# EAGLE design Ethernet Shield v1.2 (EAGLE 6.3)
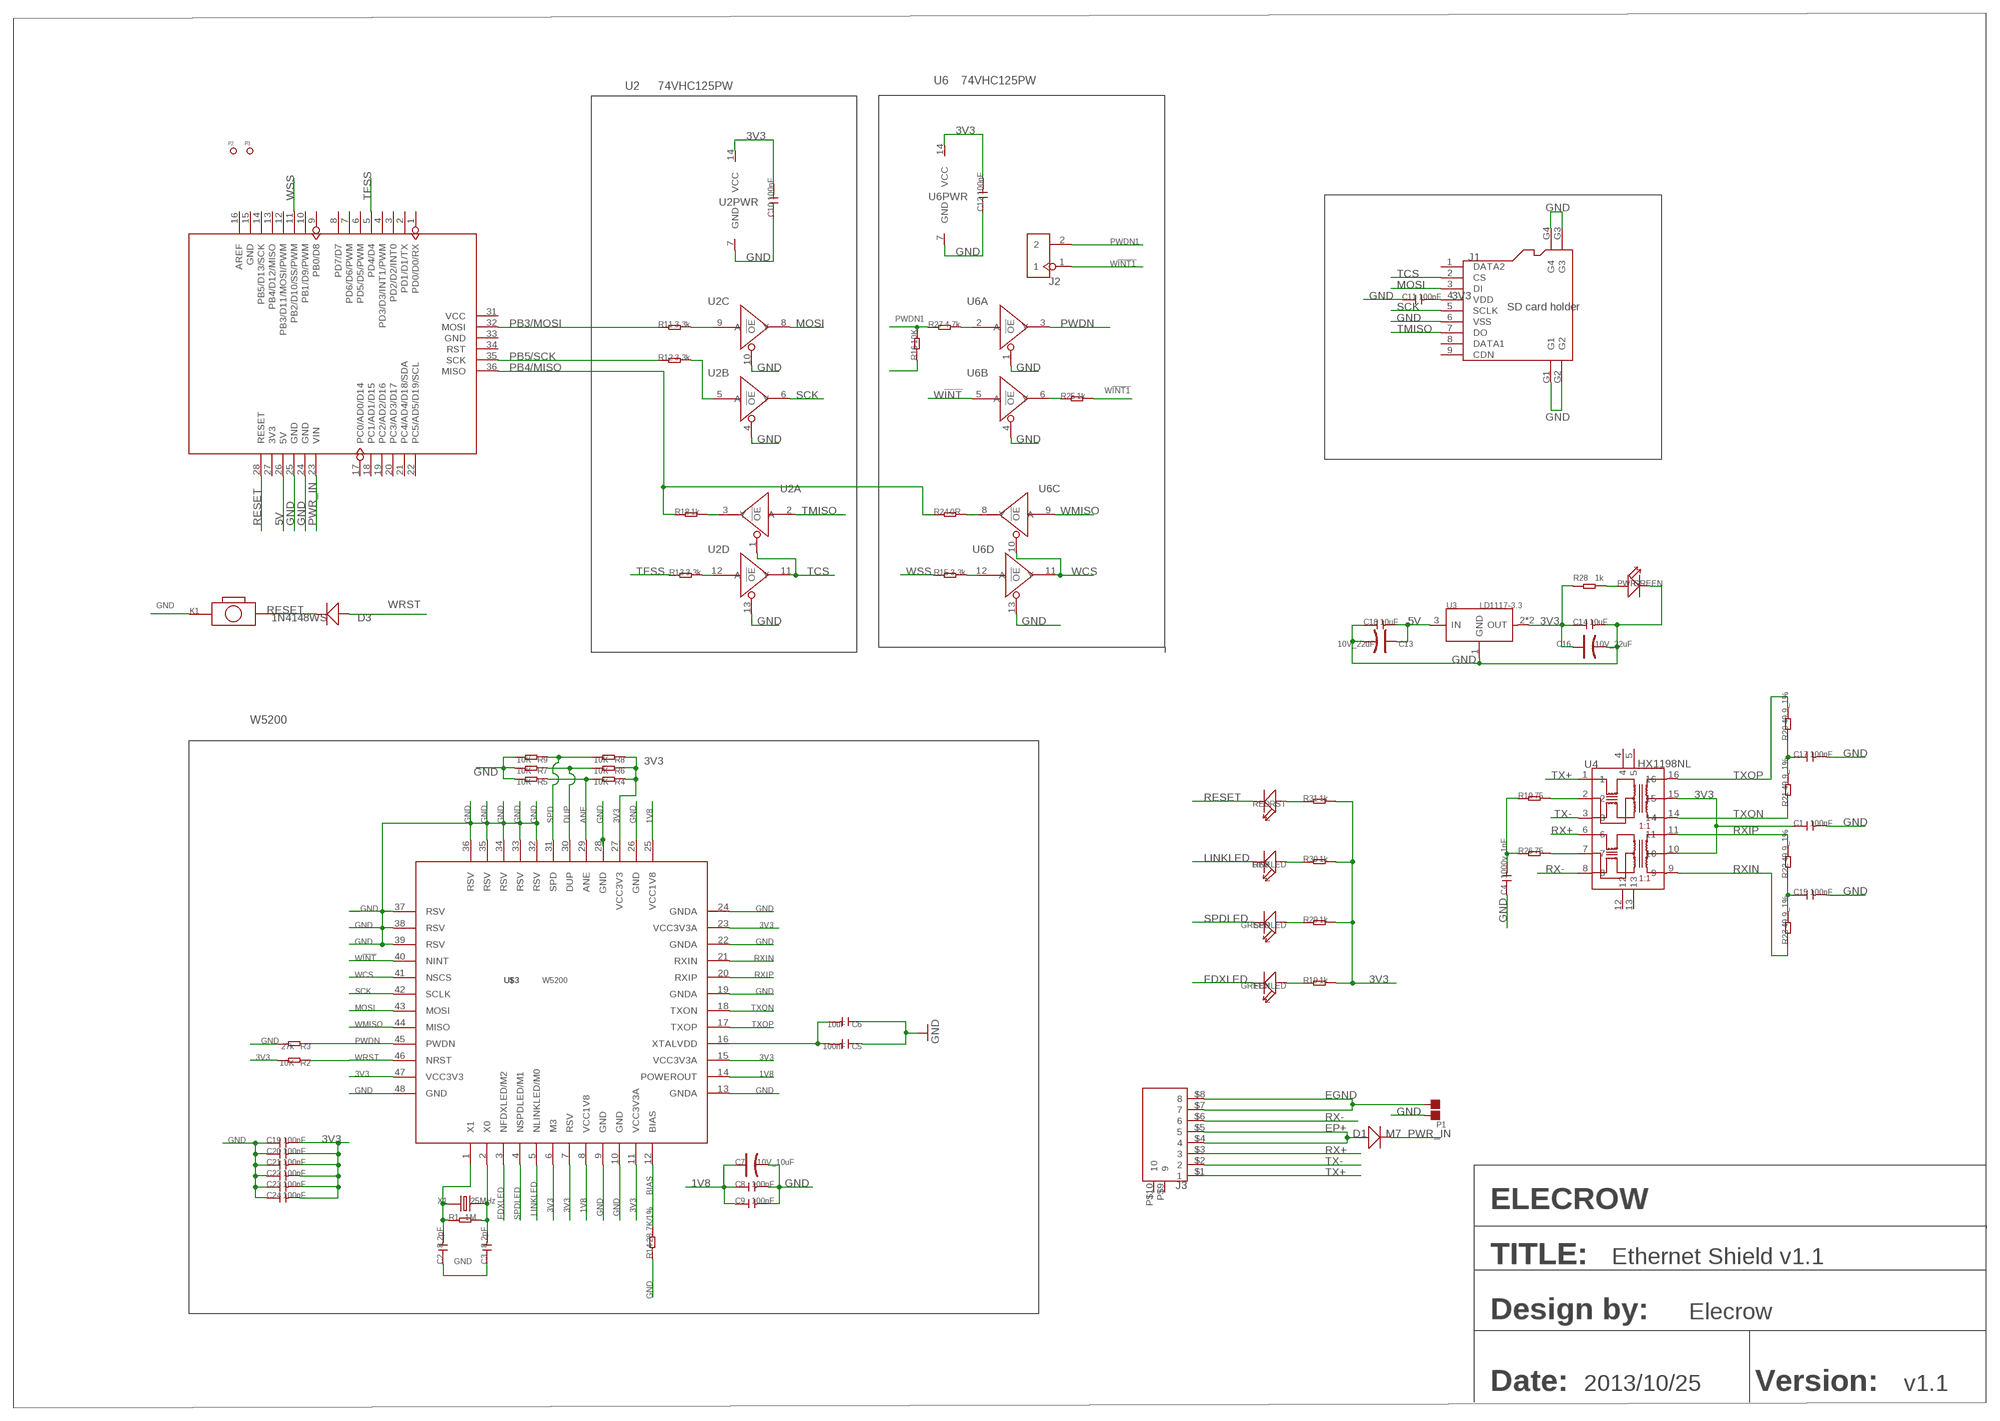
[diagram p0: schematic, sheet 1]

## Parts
C1  100nF  C-0603  [C0603]
C2  8.2pF  C-0603  [C0603]
C3  8.2pF  C-0603  [C0603]
C4  1000v_1nF  C-1206  [C1206]
C5  100nF  C-0603  [C0603]
C6  10uF  C-0805  [C0805]
C7  10V_10uF  CAP-AVX-A  [AVX-A]
C8  100nF  C-0603  [C0603]
C9  100nF  C-0603  [C0603]
C10  100nF  C-0603  [C0603]
C11  100nF  C-0603  [C0603]
C12  100nF  C-0603  [C0603]
C13  10V_22uF  CAP-AVX-B  [AVX-B]
C14  10uF  C-0805  [C0805]
C15  100nF  C-0603  [C0603]
C16  10V_22uF  CAP-AVX-B  [AVX-B]
C17  100nF  C-0603  [C0603]
C18  10uF  C-0805  [C0805]
C19  100nF  C-0805  [C0805]
C20  100nF  C-0805  [C0805]
C21  100nF  C-0805  [C0805]
C22  100nF  C-0805  [C0805]
C23  100nF  C-0805  [C0805]
C24  100nF  C-0805  [C0805]
D1  M7  D'SMA'  [D2010]
D3  1N4148WS  D'0805'  [SOD323]
FDXLED  GREEN  LED'0603'  [LED-0603]
J1  SD card holder  HOLDER-MICROSD-9P  [9P-SMD-W/-RING]
J2  HEADER-2P-65/35MIL  [2P-2.54-65/35MIL]
J3  RJ45-SMD  [RJ45_SMD]
K1  BOTTON-2P-90D  [2P-7.62X3.56-90D]
LINKLED  RED  LED'0603'  [LED-0603]
P1  DNP  PAD-JUMPER-2P  [2P-SMD-1.78X1.27]
P2  PAD-MARK  [ROUND-MARK-1.0]
P3  PAD-MARK  [ROUND-MARK-1.0]
PWR  GREEN  LED'0603'  [LED-0603]
R1  1M  R-0603  [R0603]
R2  10K  R-0603  [R0603]
R3  27k  R-0603  [R0603]
R4  10K  R-0603  [R0603]
R5  10K  R-0603  [R0603]
R6  10K  R-0603  [R0603]
R7  10K  R-0603  [R0603]
R8  10K  R-0603  [R0603]
R9  10K  R-0603  [R0603]
R10  1k  R-0603  [R0603]
R11  3.3k  R-0603  [R0603]
R12  3.3k  R-0603  [R0603]
R13  3.3k  R-0603  [R0603]
R14  28.7K/1%  R-0603  [R0603]
R15  3.3k  R-0603  [R0603]
R16  10K  R-0603  [R0603]
R18  1k  R-0603  [R0603]
R19  75  R-0603  [R0603]
R20  49.9_1%  R-0603  [R0603]
R21  49.9_1%  R-0603  [R0603]
R22  49.9_1%  R-0603  [R0603]
R23  49.9_1%  R-0603  [R0603]
R24  0R  R-0603  [R0603]
R25  1k  R-0603  [R0603]
R26  75  R-0603  [R0603]
R27  4.7k  R-0603  [R0603]
R28  1k  R-0603  [R0603]
R29  1k  R-0603  [R0603]
R30  1k  R-0603  [R0603]
R31  1k  R-0603  [R0603]
RST  RED  LED'0603'  [LED-0603]
SPDLED  GREEN  LED'0603'  [LED-0603]
U1  ARDUINO  [ARDUINO]
U2  74VHC125PW  [TSSOP14]
U3  LD1117-3.3  LD1117S  [SOT-223]
U4  HX1198NL  [SOIC16-9.53]
U6  74VHC125PW  [TSSOP14]
U$3  W5200  [QFN48]
X1  25MHz  CRYSTAL'5032'  [2P-SMD-5X3.2]

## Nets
1V8: C7.+ C8.1 C9.1 U$3.8(VCC1V8) U$3.14(POWEROUT) U$3.25(VCC1V8)
3V3: C1.1 C10.2 C11.2 C12.2 C14.1 C16.+ C19.2 C20.2 C21.2 C22.2 C23.2 C24.2 J1.4(VDD) R2.2 R4.1 R6.1 R8.1 R10.2 R28.1 R29.2 R30.2 R31.2 U2.14(PWR:VCC) U3.2(OUT) U3.TER(OUT) U4.10 U4.15 U6.14(PWR:VCC) U$3.6(M3) U$3.7(RSV) U$3.11(VCC3V3A) U$3.15(VCC3V3A) U$3.23(VCC3V3A) U$3.27(VCC3V3) U$3.47(VCC3V3)
5V [usbvcc]: C13.+ C18.2 U1.26(5V) U3.3(IN)
ANE: R4.2 R5.1 U$3.29(ANE)
BIAS: R14.2 U$3.12(BIAS)
DUP: R6.2 R7.1 U$3.30(DUP)
EGND [power]: J3.$7 J3.$8 P1.1
EP+: D1.+ J3.$4 J3.$5
FDXLED: FDXLED.- U$3.3(NFDXLED/M2)
GND: C1.2 C2.1 C3.1 C4.1 C5.1 C6.1 C7.- C8.2 C9.2 C10.1 C11.1 C12.1 C13.- C14.2 C15.2 C16.- C17.2 C18.1 C19.1 C20.1 C21.1 C22.1 C23.1 C24.1 J1.6(VSS) J1.G1 J1.G2 J1.G3 J1.G4 K1.P$1 P1.2 PWR.- R3.2 R5.2 R7.2 R9.2 R14.1 R16.1 U1.24(GND) U1.25(GND) U2.4(B:!OE) U2.7(PWR:GND) U2.10(C:!OE) U2.13(D:!OE) U3.1(GND) U6.1(A:!OE) U6.4(B:!OE) U6.7(PWR:GND) U6.13(D:!OE) U$3.9(GND) U$3.10(GND) U$3.13(GNDA) U$3.19(GNDA) U$3.22(GNDA) U$3.24(GNDA) U$3.26(GND) U$3.28(GND) U$3.32(RSV) U$3.33(RSV) U$3.34(RSV) U$3.35(RSV) U$3.36(RSV) U$3.37(RSV) U$3.38(RSV) U$3.39(RSV) U$3.48(GND)
LINKLED: LINKLED.- U$3.5(NLINKLED/M0)
MOSI: J1.3(DI) U2.8(C:Y) U$3.43(MOSI)
N$1: R29.1 SPDLED.+
N$2: LINKLED.+ R30.1
N$3: R31.1 RST.+
N$6: FDXLED.+ R10.1
N$7: R12.2 U2.5(B:A)
N$8: R11.2 U2.9(C:A)
N$9: R13.2 U2.12(D:A)
N$10: R15.2 U6.12(D:A)
N$11: R26.2 U4.7
N$12: R19.2 U4.2
N$13: C4.2 R19.1 R26.1
N$14: R18.2 U2.3(A:Y)
N$15: C15.1 R22.1 R23.2
N$16: C17.1 R20.1 R21.2
N$17: R24.2 U6.8(C:Y)
N$20: R25.1 U6.6(B:Y)
N$24: R27.2 U6.2(A:A)
N$26: PWR.+ R28.2
PB3/MOSI: R11.1 U1.32(MOSI)
PB4/MISO: R18.1 R24.1 U1.36(MISO)
PB5/SCK: R12.1 U1.35(SCK)
PWDN: R3.1 U6.3(A:Y) U$3.45(PWDN)
PWDN1: J2.2 R16.2 R27.1
PWR_IN: D1.- U1.23(VIN)
RESET: D3.- K1.P$2 RST.- U1.28(RESET)
RX+: J3.$3 U4.6
RX-: J3.$6 U4.8
RXIN: R23.1 U4.9 U$3.21(RXIN)
RXIP: R22.2 U4.11 U$3.20(RXIP)
SCK: J1.5(SCLK) U2.6(B:Y) U$3.42(SCLK)
SPD: R8.2 R9.1 U$3.31(SPD)
SPDLED: SPDLED.- U$3.4(NSPDLED/M1)
TCS: J1.2(CS) U2.1(A:!OE) U2.11(D:Y)
TFSS: R13.1 U1.5(PD4/D4)
TMISO: J1.7(DO) U2.2(A:A)
TX+: J3.$1 U4.1
TX-: J3.$2 U4.3
TXON: R21.1 U4.14 U$3.18(TXON)
TXOP: R20.2 U4.16 U$3.17(TXOP)
W!INT: U6.5(B:A) U$3.40(NINT)
W!INT1: J2.1 R25.2
WCS: U6.10(C:!OE) U6.11(D:Y) U$3.41(NSCS)
WMISO: U6.9(C:A) U$3.44(MISO)
WRST: D3.+ R2.1 U$3.46(NRST)
WSS: R15.1 U1.11(PB2/D10/SS/PWM)
X0: C3.2 R1.2 U$3.2(X0) X1.2
X1: C2.2 R1.1 U$3.1(X1) X1.1
XTALVDD: C5.2 C6.2 U$3.16(XTALVDD)
Unconnected: J1.1(DATA2) J1.8(DATA1) J1.9(CDN) J3.P$9 J3.P$10 U1.1(PD0/D0/RX) U1.2(PD1/D1/TX) U1.3(PD2/D2/INT0) U1.4(PD3/D3/INT1/PWM) U1.6(PD5/D5/PWM) U1.7(PD6/D6/PWM) U1.8(PD7/D7) U1.9(PB0/D8) U1.10(PB1/D9/PWM) U1.12(PB3/D11/MOSI/PWM) U1.13(PB4/D12/MISO) U1.14(PB5/D13/SCK) U1.15(GND) U1.16(AREF) U1.17(PC0/AD0/D14) U1.18(PC1/AD1/D15) U1.19(PC2/AD2/D16) U1.20(PC3/AD3/D17) U1.21(PC4/AD4/D18/SDA) U1.22(PC5/AD5/D19/SCL) U1.27(3V3) U1.31(VCC) U1.33(GND) U1.34(RST) U4.4 U4.5 U4.12 U4.13

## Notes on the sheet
- U6 | 74VHC125PW
- U2 | 74VHC125PW
- W5200
- ELECROW
- TITLE: | TITLE: | Ethernet Shield v1.1
- Design by: | Elecrow
- Date: | 2013/10/25 | Version: | v1.1

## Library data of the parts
C1-C6 C8-C12 C14 C15 C17-C24 = Discrete:C*: Ceramic Capacitors
C7 C13 C16 = Discrete:CAP*: Electrolytic Capacitors,Tantalum Capacitors and Super Capacitors
D1 D3 = Discrete:D*
FDXLED LINKLED PWR RST SPDLED = Discrete:LED*
J1 = Connector:HOLDER-MICROSD-9P
J2 = Connector:HEADER-2P
J3 = Elecrow_test:RJ45-SMD: Modular Jack 8P8C,R/A,With LED
K1 = Discrete:BOTTON-2P
P1 = Discrete:PAD-JUMPER-2P; PARTNO: DNP
P2 P3 = Discrete:PAD-MARK; PARTNO: DNP
R1-R16 R18-R31 = Discrete:R*
U1 = moudle:ARDUINO
U2 U6 = IC:74V*125: Quad Buffer/Line Driver;3-state
U3 = IC:LD1117: Low Drop Fixed And Adjustable Positive Voltage Regulators http://www.datasheetcatalog.org/datasheet/SGSThomsonMicroelectronics/mXuqtqv.pdf
U4 = IC:HX1198NL: 10/100BASE-T Single Port Surface Mount Magnetics With Various Turns Ratios
U$3 = Elecrow_test:W5200
X1 = Discrete:CRYSTAL*: CRYSTAL

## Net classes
0 default: width 0.203 mm, drill 0.305 mm, clearance 0.152 mm
3 usbvcc: width 0.203 mm, drill 0.305 mm, clearance 0.203 mm

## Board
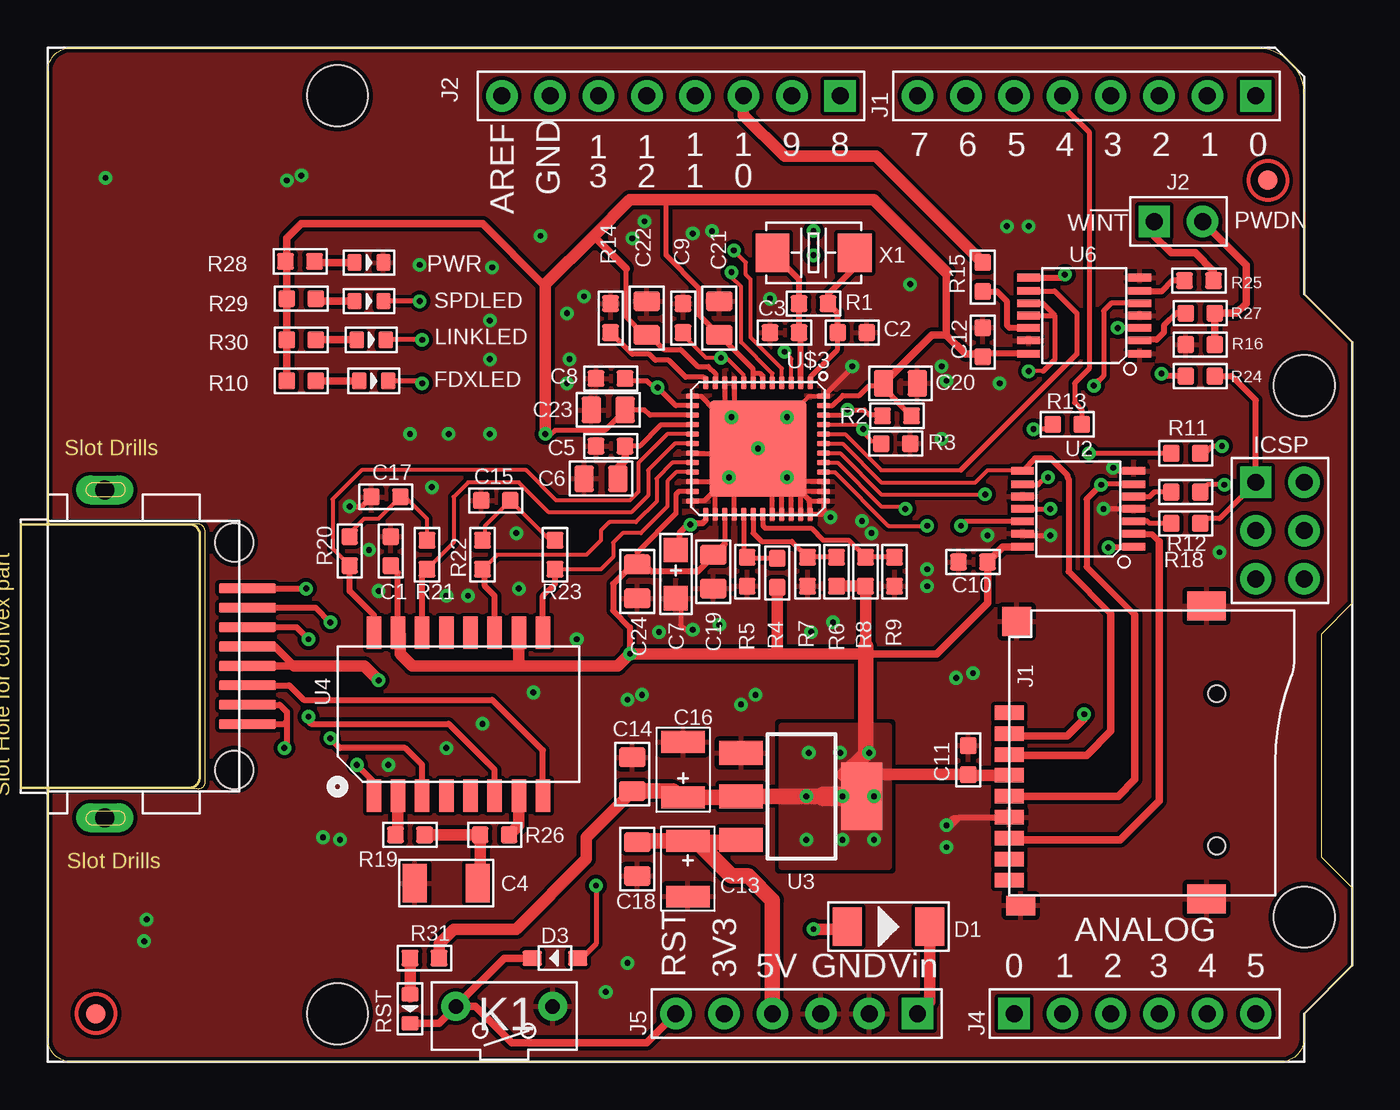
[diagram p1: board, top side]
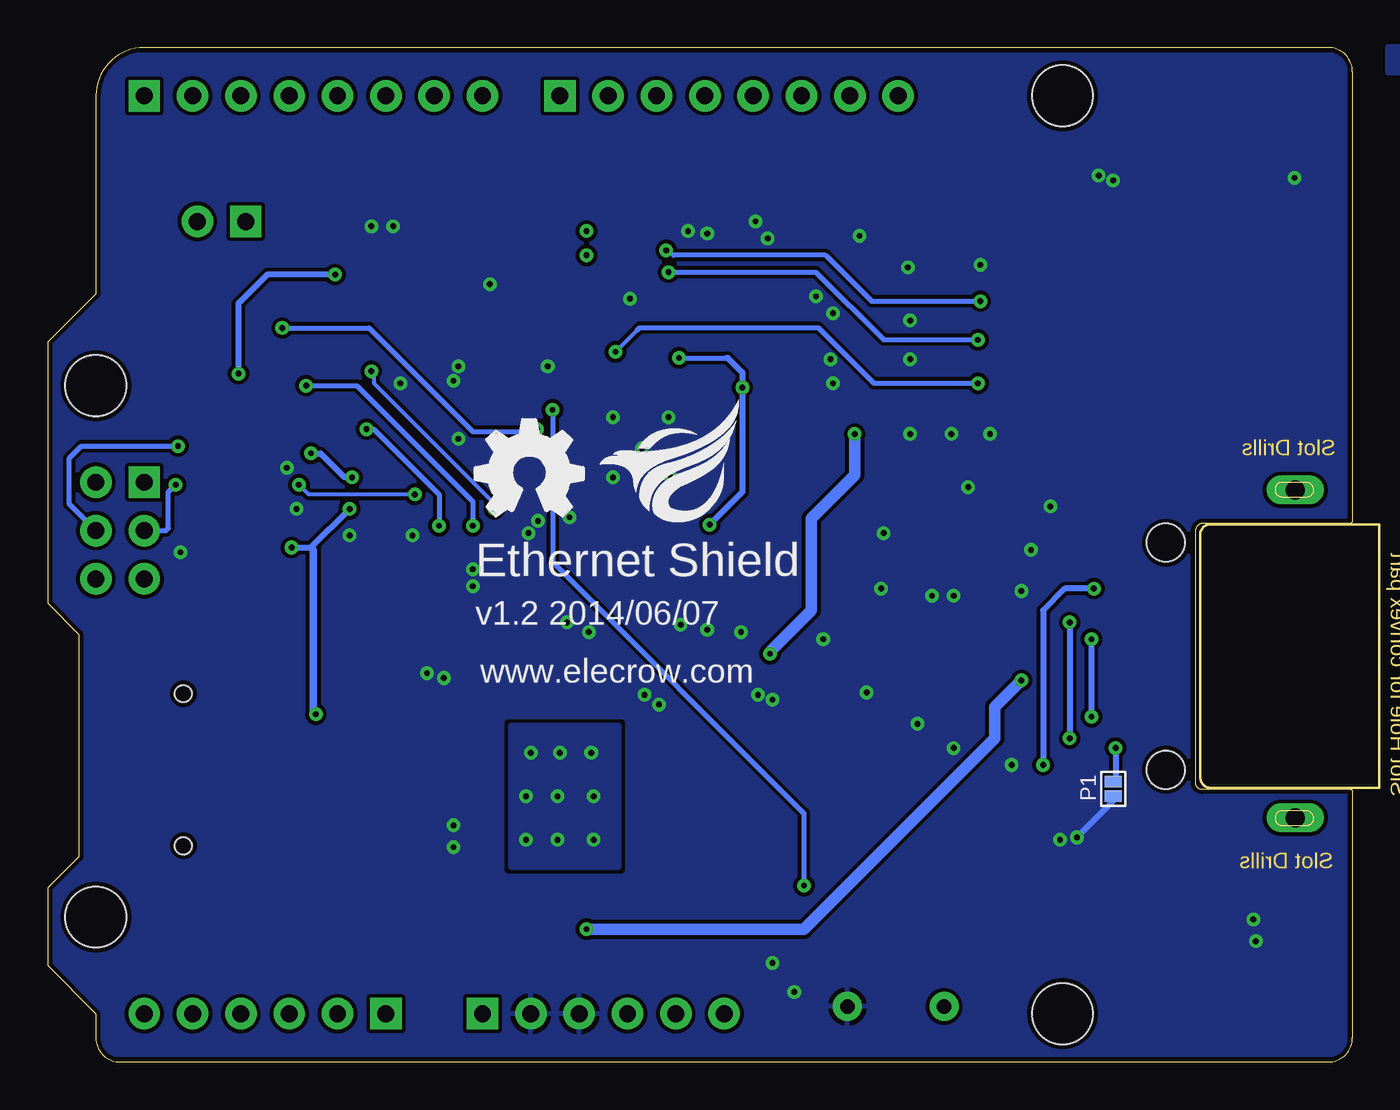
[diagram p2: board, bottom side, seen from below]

Size 68.58 x 53.34 mm. Coordinates in mm from the lower left corner, seen from the top.
Outline: 0,52.07 0,28.45 arc90 0.13,28.32 7.77,28.32 arc-90 8.26,27.96 8.26,14.63 arc-90 7.84,14.35 0.13,14.35 arc90 0,14.22 0,1.27 arc90 1.27,0 64.77,0 arc90 66.04,1.27 66.04,2.54 68.58,5.08 68.58,9.14 66.93,10.79 66.93,22.48 68.58,24.13 68.58,37.85 66.04,40.39 66.04,50.8 arc90 63.5,53.34 1.27,53.34 arc90 0,52.07
Copper layers (1*16): Top 0.035mm / dielectric 1.5mm / Bottom 0.035mm
Design rules "default *": minimum track width 8mil, minimum drill 12mil, track to track 8mil, track to pad 8mil, pad to pad 8mil, via to via 10mil, smd to smd 0mil, copper to edge 10mil, drill to drill 8mil, minimum pad ring 10mil, minimum via ring 8mil, stop-mask expansion 4mil, vias tented up to drill 25mil, thermal gap 10mil
Holes 3.2 mm at 15.24,2.54

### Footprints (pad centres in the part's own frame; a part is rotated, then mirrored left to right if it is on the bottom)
C0603 = smd 0.889 x 0.889: 1 -0.762,0; 2 0.762,0
C1206 = smd 1.27 x 2.032: 1 -1.651,0; 2 1.651,0
C0805 = smd 1.016 x 1.397: 1 -0.889,0; 2 0.889,0
AVX-A = smd 1.27 x 1.27: + -1.27,0; - 1.27,0
AVX-B = smd 1.143 x 2.286: + -1.46,0; - 1.46,0
D2010 = smd 1.524 x 2.032: + -2.159,0; - 2.159,0
SOD323 = smd 1 x 0.8: + -1.2,0; - 1.2,0
LED-0603 = smd 0.762 x 0.889: + -0.762,0; - 0.762,0
9P-SMD-W/-RING = smd 1.524 x 0.762: 1 0,4.4; 2 0,3.3; 3 0,2.2; 4 0,1.1; 5 0,0; 6 0,-1.1; 7 0,-2.2; 8 0,-3.3; 9 0,-4.4 | smd 1.524 x 1.016: G1 0.6,-5.746 | smd 2.032 x 1.524: G2 10.373,-5.4; G3 10.373,10 | smd 1.524 x 1.524: G4 0.392,9.181 | hole 0.889: 10.9,-2.6; 10.9,5.4
2P-2.54-65/35MIL = drill 0.889 pad 1.651 square: 1 0,1.27 | drill 0.889 pad 1.651: 2 0,-1.27
RJ45_SMD = smd 0.5 x 3: $1 -3.57,10.5; $2 -2.55,10.5; $3 -1.53,10.5; $4 -0.51,10.5; $5 0.51,10.5; $6 1.53,10.5; $7 2.55,10.5; $8 3.57,10.5 | drill 1 pad 1.511 long: P$9 8.493,3; P$10 -8.747,3 | hole 2: -5.97,9.8; 5.97,9.8
2P-7.62X3.56-90D = drill 0.762 pad 1.524: P$1 0,2.54; P$2 0,-2.54
2P-SMD-1.78X1.27 = smd 0.889 x 0.61: 1 0,0.381; 2 0,-0.381
ROUND-MARK-1.0 = smd 1.016 x 1.016: P$1 0,0
R0603 = smd 0.889 x 0.889: 1 -0.762,0; 2 0.762,0
ARDUINO = drill 0.889 pad 1.651 square: 1 63.5,50.8; 9 41.656,50.8; 17 50.8,2.54; 23 45.72,2.54; 36 63.5,30.48 | drill 0.889 pad 1.651: 2 60.96,50.8; 3 58.42,50.8; 4 55.88,50.8; 5 53.34,50.8; 6 50.8,50.8; 7 48.26,50.8; 8 45.72,50.8; 10 39.116,50.8; 11 36.576,50.8; 12 34.036,50.8; 13 31.496,50.8; 14 28.956,50.8; 15 26.416,50.8; 16 23.876,50.8; 18 53.34,2.54; 19 55.88,2.54; 20 58.42,2.54; 21 60.96,2.54; 22 63.5,2.54; 24 43.18,2.54; 25 40.64,2.54; 26 38.1,2.54; 27 35.56,2.54; 28 33.02,2.54; 31 66.04,30.48; 32 66.04,27.94; 33 66.04,25.4; 34 63.5,25.4; 35 63.5,27.94 | hole 3.2: 15.24,50.8; 66.04,35.56; 66.04,7.62
TSSOP14 = smd 0.4 x 1.2: 1 -2,-2.925; 2 -1.3,-2.925; 3 -0.65,-2.925; 4 0,-2.925; 5 0.65,-2.925; 6 1.3,-2.925; 7 2,-2.925; 8 2,2.925; 9 1.3,2.925; 10 0.65,2.925; 11 0,2.925; 12 -0.65,2.925; 13 -1.3,2.925; 14 -2,2.925
SOT-223 = smd 1.27 x 2.286: 1 -2.286,-3.175; 2 0,-3.175; 3 2.286,-3.175 | smd 3.556 x 2.159: TER 0,3.175
SOIC16-9.53 = smd 0.762 x 1.714: 1 -4.445,-4.286; 2 -3.175,-4.286; 3 -1.905,-4.286; 4 -0.635,-4.286; 5 0.635,-4.286; 6 1.905,-4.286; 7 3.175,-4.286; 8 4.445,-4.286; 9 4.445,4.286; 10 3.175,4.286; 11 1.905,4.286; 12 0.635,4.286; 13 -0.635,4.286; 14 -1.905,4.286; 15 -3.175,4.286; 16 -4.445,4.286
QFN48 = smd 0.3 x 0.7: 1 -2.369,-2.815; 2 -1.869,-2.815; 3 -1.369,-2.815; 4 -0.869,-2.815; 5 -0.369,-2.815; 6 0.131,-2.815; 7 0.631,-2.815; 8 1.131,-2.815; 9 1.631,-2.815; 10 2.131,-2.815; 11 2.631,-2.815; 12 3.131,-2.815; 25 3.131,4.085; 26 2.631,4.085; 27 2.131,4.085; 28 1.631,4.085; 29 1.131,4.085; 30 0.631,4.085; 31 0.131,4.085; 32 -0.369,4.085; 33 -0.869,4.085; 34 -1.369,4.085; 35 -1.869,4.085; 36 -2.369,4.085 | smd 0.7 x 0.3: 13 3.831,-2.115; 14 3.831,-1.615; 15 3.831,-1.115; 16 3.831,-0.615; 17 3.831,-0.115; 18 3.831,0.385; 19 3.831,0.885; 20 3.831,1.385; 21 3.831,1.885; 22 3.831,2.385; 23 3.831,2.885; 24 3.831,3.385; 37 -3.069,3.385; 38 -3.069,2.885; 39 -3.069,2.385; 40 -3.069,1.885; 41 -3.069,1.385; 42 -3.069,0.885; 43 -3.069,0.385; 44 -3.069,-0.115; 45 -3.069,-0.615; 46 -3.069,-1.115; 47 -3.069,-1.615; 48 -3.069,-2.115 | smd 5.1 x 5.1: PAD 0.381,0.635
2P-SMD-5X3.2 = smd 1.778 x 2.032: 1 -2.159,0; 2 2.159,0

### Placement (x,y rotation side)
C1  18.03,26.86 90 top
C2  42.29,38.35 180 top
C3  38.73,38.35 0 top
C4  20.95,9.4 0 top
C5  29.59,32.38 0 top
C6  29.08,30.67 0 top
C7  33.02,25.65 270 top
C8  29.59,35.94 180 top
C9  33.4,39.12 90 top
C10  48.64,26.29 0 top
C11  48.39,15.88 270 top
C12  49.15,37.85 270 top
C13  33.66,10.16 270 top
C14  30.73,15.14 90 top
C15  23.56,29.53 180 top
C16  33.4,15.37 90 top
C17  17.78,29.72 180 top
C18  30.99,10.67 90 top
C19  34.99,25.78 90 top
C20  44.83,35.69 180 top
C21  35.31,39.12 270 top
C22  31.5,39.12 270 top
C23  29.46,34.29 0 top
C24  30.99,25.27 90 top
D1  44.2,7.11 0 top
D3  26.67,5.46 180 top
FDXLED  17.14,35.81 0 top
J1  50.55,13.97 0 top
J2  59.44,44.2 90 top
J3  0,21.34 270 top
K1  24,2.92 270 top
LINKLED  17.02,37.97 0 top
P1  12.57,14.35 0 bottom
P2  2.54,2.54 0 top
P3  64.14,46.35 0 top
PWR  16.89,42.04 0 top
R1  40.26,39.88 180 top
R2  44.64,33.97 0 top
R3  44.58,32.51 0 top
R4  38.35,25.72 90 top
R5  36.77,25.78 270 top
R6  41.47,25.78 90 top
R7  39.94,25.78 270 top
R8  42.99,25.78 90 top
R9  44.51,25.78 270 top
R10  13.34,35.81 180 top
R11  59.82,32 180 top
R12  59.82,29.97 180 top
R13  53.59,33.53 180 top
R14  29.59,39.12 270 top
R15  49.15,41.27 270 top
R16  60.58,37.72 0 top
R18  59.82,28.32 180 top
R19  19.05,11.94 180 top
R20  15.88,26.86 270 top
R21  19.94,26.67 90 top
R22  22.86,26.67 270 top
R23  26.67,26.67 90 top
R24  60.58,36.07 180 top
R25  60.52,41.08 0 top
R26  23.5,11.94 0 top
R27  60.58,39.37 180 top
R28  13.27,42.1 0 top
R29  13.34,40.13 180 top
R30  13.34,37.97 180 top
R31  19.81,5.46 0 top
RST  19.05,2.79 270 top
SPDLED  16.89,40.01 0 top
U1  0,0 0 top
U2  54.17,29.08 90 top
U3  39.62,13.97 270 top
U4  21.59,18.29 0 top
U6  54.48,39.24 90 top
U$1  [ELECROW_NRW_6]  39.56,28.38 0 bottom
U$2  [OSHW_FILLX200_NOTEXT]  46.1,28.7 0 bottom
U$3  37.72,32.89 180 top
X1  40.26,42.55 180 top

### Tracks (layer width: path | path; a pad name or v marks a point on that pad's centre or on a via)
1V8  (via drill 0.3)
  Top 0.203: U$3.8 36.59,36.12 35.69,37.02 v35.4,37.02 34.61,37.02 33.4,38.23 C9.1
  Top 0.254: C8.1 30.48,35.81 31.5,35.81 31.85,35.46 v32.07,35.46 33.02,34.51 U$3.14 | U$3.25 34.59,28.49
  Top 0.305: 34.59,28.49 34.42,28.32 33.85,28.32 v33.78,28.26 33.66,28.26 33.21,27.81 33.21,27.11 C7.+
  Bottom 0.254: v35.4,37.02 32.89,37.02
  Bottom 0.305: 32.89,37.02 32.83,37.02 32.07,36.26 v32.07,35.46 32.07,29.97 v33.78,28.26
3V3  (via drill 0.3)
  Top 0.254: U$3.6 37.59,36.07 37.47,36.2 37.09,36.2 | U$3.7 37.09,36.2 | 37.09,36.2 37.09,36.45 C21.2 34.23,39.31 34.23,40.7 32.51,42.42 32.51,45.34 | U$3.23 33.18,30.01 33.02,29.84 33.02,28.83 30.99,26.8 C24.2 30.99,26.42 31.11,26.54 | 30.67,33.97 30.61,34.04 | 30.61,34.04 C23.2 | U$3.27 35.59,27.27 C19.2 | R2.2 43.94,35.43 C20.2 43.81,35.56 43.18,35.56 42.67,35.05 41.78,35.05 41.24,34.51 U$3.47 | 30.61,34.04 30.61,33.78 | 26.29,33.15 v26.16,33.02 26.48,33.02 26.67,33.21 29.27,33.21 C23.2 | C23.2 31.37,34.29 31.65,34.01 U$3.15 | 31.75,25.78 31.37,26.16 | 26.29,39.12 26.16,39.24 | 30.42,41.72 30.42,39.18 31.37,38.23 C22.2 31.62,38.23 32.38,37.47 33.27,37.47 34.16,36.58 34.73,36.58 35.12,36.2 35.12,35.74 U$3.11 35.05,35.74
  Top 0.305: U6.14 49.31,37.24 C12.2 49.02,36.96 | 35.59,27.27 35.59,27.21 34.16,25.78 31.75,25.78 | 31.37,26.54 31.11,26.54 29.72,25.15 29.72,23.75 30.61,22.86 v30.61,21.46 | U4.15 18.41,25.72 C1.1 | 31.37,26.16 C24.2
  Top 0.406: 30.42,41.72 28.7,43.43 | 47.24,41.53 47.24,38.23 | 47.24,38.23 48.26,37.21 49.02,37.21 C12.2 | 47.24,38.23 46.48,38.23 C20.2 | 26.16,40.89 26.04,40.89 22.86,44.07 13.34,44.07 12.57,43.31 12.57,42.16 R28.1 12.57,42.04 R29.2 R30.2 R10.2 | U2.14 50.2,27.08 C10.2 49.4,24.13 46.74,21.46 43.18,21.46
  Top 0.61: 38.35,21.46 43.18,21.46 42.99,21.65 42.99,21.84 R8.1 R6.1 | 38.35,21.46 v30.61,21.46 29.97,20.83 24.77,20.83 | R4.1 38.35,21.46 | U4.15 18.54,22.45 18.54,21.46 19.18,20.83 24.77,20.83 | U4.10 24.77,20.83 | J1.4 48.43,15.07 C11.2 41.91,15.11 | v26.16,33.02 26.16,39.24 26.16,40.89 28.7,43.43 30.61,45.34 32.51,45.34 43.43,45.34 47.24,41.53 | C14.1 30.73,14.22 28.32,11.81 28.32,10.67 24.64,6.99 21.34,6.99 20.57,6.22 R31.2
  Top 0.813: 41.91,15.11 42.99,16.19 42.99,21.84 | 40.77,13.97 v39.88,13.97 U3.2 36.39,13.91 C16.+ 33.34,13.97 32.77,13.97 32.89,13.84 33.27,13.84 32.87,14.25 C14.1
  Top 1.016: 40.77,13.97 U3.TER
  Bottom 0.61: v30.61,21.46 30.61,21.59 28.45,23.75 28.45,28.57 26.16,30.86 v26.16,33.02
  other vias: 40.01,16.26 39.88,11.68 41.78,11.68 43.43,11.68 41.78,13.97 43.43,13.97 41.66,16.26 43.18,16.26
  pour Top (isolate 0.406, no thermals): 38.61,10.29 44.2,10.29 44.2,17.65 38.61,17.65
  pour Bottom (isolate 0.406, no thermals): 38.61,10.29 44.2,10.29 44.2,17.65 38.61,17.65
5V
  Top 0.813: U1.26 38.1,8.51 36.83,9.78 35.94,9.78 34.16,11.56 33.72,11.56 C13.+ | C13.+ 34.35,11.62 34.42,11.56 36.32,11.56 U3.3 | C13.+ 31.05,11.62 C18.2
ANE
  Top 0.254: 36.52,26.79 R5.1 | U$3.29 36.59,26.72 R5.1 | R4.2 36.83,26.48 R5.1
BIAS
  Top 0.254: U$3.12 34.59,35.9 34.48,36.01 33.53,36.01 32.64,36.89 31.94,36.89 31.62,37.21 30.73,37.21 R14.2
DUP
  Top 0.254: U$3.30 37.09,27.81 37.53,27.37 39.12,27.37 R7.1 R6.2
EGND  (via drill 0.3)
  Top 0.305: J3.$8 12.43,17.77 12.57,17.91 | J3.$7 12.2,18.79 12.57,18.41 12.57,17.91 | 12.57,17.91 12.57,16.64 v12.45,16.51
  Bottom 0.305: v12.45,16.51 12.45,14.86 P1.1
EP+  (via drill 0.3)
  Top 0: v17.4,20.07 v17.39,20.07
  Top 0.406: J3.$5 12.95,20.83 11.93,21.85 J3.$4 | 16.64,20.83
  Top 0.61: D1.+ 41.91,6.99 v40.26,6.99 | 12.95,20.83 16.64,20.83 v17.4,20.07
  Bottom 0.61: v40.26,6.99 28.83,6.99 18.8,17.02 18.8,18.67 v17.4,20.07
FDXLED  (via drill 0.3)
  Top 0.203: U$3.3 39.09,36.98 v38.73,37.34
  Top 0.254: v19.68,35.69 19.56,35.81 FDXLED.-
  Bottom 0.203: v38.73,37.34 37.59,38.48
  Bottom 0.254: 37.59,38.48 37.47,38.61 28.07,38.61 25.15,35.69 v19.68,35.69
GND  (via drill 0.3)
  Top 0.203: U$3.48 40.77,34.99 40.01,34.99 38.92,33.91 v38.86,33.91
  Top 0.254: v38.86,33.91 38.99,33.91 | U$3.48 42.29,36.51 v42.29,36.58 | v15.88,29.21 16.51,29.21 C17.2 | U$3.9 36.09,33.91 v35.94,33.91 35.59,34.26 | U$3.10 35.59,34.26 | U$3.13 34.33,35.01 35.05,34.29 35.56,34.29 35.59,34.26 | U$3.22 35.59,30.51 v35.81,30.73 | U$3.26 35.09,30.01 | 35.09,30.01 v35.81,30.73 | U$3.28 36.09,30.73 v35.81,30.73 | U$3.32 38.09,29.96 v38.86,30.73 | U$3.33 38.59,30.46 v38.86,30.73 | U$3.34 39.09,30.51 | U$3.35 39.59,30.01 | 39.59,30.01 v38.86,30.73 | U$3.38 39.59,30.01 | U$3.39 39.09,30.51 | 39.09,30.51 v38.86,30.73 | v38.86,30.73 40.07,29.53 | 40.07,29.53 40.09,29.51 U$3.37 40.79,29 v41.15,28.64 40.98,28.81 U$3.36 40.07,28.83 40.07,29.53 | 35.09,30.01 34.96,30.01 34.96,29.95 34.54,29.53 33.91,29.53 U$3.24 | U2.4 v55.5,29.08 | U2.13 51.34,27.69 v52.7,27.69 | C7.- 33.27,24.13 33.27,22.99 33.53,22.73 v33.91,22.73 | U$3.19 36.2,32 36.45,32.26 v37.34,32.26 | U2.7 56.17,31.08 v56.01,31.24
  Top 0.305: J1.6 50.5,12.83 47.88,12.83 | 47.88,12.83 47.5,12.45 v47.24,12.45 47.62,12.83 47.88,12.83
  Bottom 0.305: P1.2 12.57,13.72 v14.48,11.81
  other vias: 46.99,36.58 47.24,35.81 42.8,28.45 43.31,27.81 46.23,25.91 46.23,25.02 41.27,23.11 40.13,22.61 35.31,22.99 15.37,11.68 23.24,36.96 19.05,33.02 21.08,33.02 31.37,44.2 30.73,43.31 28.19,40.26 27.3,39.37 27.43,36.96 27.3,35.69 20.95,24.51 22.1,24.51 20.19,30.23 17.4,24.77 17.91,15.62 29.34,3.68 30.48,5.21 16.89,26.92 23.24,33.02 30.48,19.05 31.24,19.3 20.95,16.51 22.86,17.78 25.53,19.43 47.24,11.3 47.75,20.19 48.64,20.45 46.99,32.77 50.04,35.69 33.91,43.56 34.92,43.69 45.34,40.89 37.97,40.13 32.13,22.61 23.24,38.99 23.37,41.78 19.56,41.91 5.21,7.49 3.05,46.48 37.21,19.3 5.08,6.35 13.34,46.61 36.45,18.8 61.59,26.8 50.42,43.94 51.56,43.94 25.91,43.43 12.57,46.35 49.4,27.69 24.77,24.89 24.64,27.81 27.81,22.23
  pour Bottom: -3.17,53.34 -1.91,53.34 -1.91,52.07 -3.17,52.07
  pour Top (rank 6): 0,53.34 68.96,53.34 68.96,0 68.96,-0.13 0,-0.13
  pour Bottom (isolate 0.152, rank 6): 0,53.34 68.83,53.34 68.83,-0.13 0,-0.13
LINKLED  (via drill 0.3)
  Top 0.203: U$3.5 38.09,36.21 36.45,37.85 36.45,40.77 35.94,41.27 v35.94,41.53
  Top 0.254: v19.68,37.97 LINKLED.-
  Bottom 0.254: v19.68,37.97 24.64,37.97 28.19,41.53 v35.94,41.53
MOSI
  Top 0.203: U$3.43 41.79,32.51 43.81,30.48 48.77,30.48 49.4,31.11 50.16,31.11 50.67,31.11 51.21,31.11 U2.8
  Top 0.305: U2.8 51.91,31.75 52.7,31.75 53.59,30.86 53.59,30.73 53.66,30.67 53.66,25.78 55.88,23.56
  Top 0.406: J1.3 50.59,16.13 54.61,16.13 55.88,17.4 55.88,23.56
N$1
  Top 0.406: R29.1 14.22,40.01 SPDLED.+
N$2
  Top 0.406: R30.1 LINKLED.+
N$3
  Top 0.61: R31.1 RST.+ 19.05,3.43
N$6
  Top 0.406: R10.1 FDXLED.+
N$7
  Top 0.254: R12.2 58.17,29.97 57.91,29.72 57.1,29.72 U2.5
N$8  (via drill 0.3)
  Top 0.254: R11.2 v54.74,32 | U2.9 51.27,30.35 52.07,30.35 52.45,30.73 v52.58,30.73
  Bottom 0.305: v54.74,32 54.23,32 52.96,30.73 v52.58,30.73
N$9  (via drill 0.3)
  Top 0.254: 51.23,28.45 U2.12 48.24,28.43 v48.01,28.19 | R13.2 52.58,33.27 v51.82,33.27
  Bottom 0.254: v51.82,33.27 51.44,33.27 48.01,29.84 v48.01,28.19
N$10
  Top 0.305: R15.2 49.91,40.51 50.42,40.01 50.42,38.73 50.55,38.61 51.54,38.61 U6.12
N$11
  Top 0.61: U4.7 24.77,12.45 R26.2
N$12
  Top 0.61: U4.2 18.41,12.06 R19.2
N$13
  Top 0.61: R19.1 R26.1 22.73,9.53 C4.2
N$14
  Top 0.254: R18.2 57.91,28.32 57.78,28.45 57.1,28.45 U2.3
N$15
  Top 0.203: R23.2 26.42,27.43 C15.1 22.99,28.19 22.99,27.56 R22.1
N$16
  Top 0.203: R20.1 15.88,27.81 16.64,28.57 17.4,28.57 C17.1 18.8,29.72 19.94,28.57 R21.2
N$17  (via drill 0.3)
  Top 0.305: U6.8 53.31,41.24 v53.47,41.4 | R24.2 58.67,36.07 v58.55,36.2
  Bottom 0.305: v53.47,41.4 57.02,41.4 58.55,39.88 v58.55,36.2
N$20
  Top 0.305: R25.1 59.12,41.08 58.55,40.51 57.44,40.51 U6.6
N$21  (via drill 0.3)
  other vias: 40.26,43.69
N$22  (via drill 0.3)
  other vias: 40.26,42.42
N$24
  Top 0.305: R27.2 59.31,39.37 58.67,38.73 58.67,38.35 58.29,37.97 57.44,37.97 U6.2
N$26
  Top 0.406: R28.2 14.1,42.04 PWR.+
PB3/MOSI  (via drill 0.3)
  Top 0.254: 61.34,32.38 v61.72,32.38 61.21,32.38 60.83,32 R11.1
  Bottom 0.254: U1.32 67.44,29.34 67.44,31.75 66.8,32.38 v61.72,32.38
PB4/MISO
  Top 0.254: U1.36 61.59,28.57 60.83,28.57 R18.1
  Top 0.305: U1.36 63.5,34.8 62.23,36.07 R24.1
PB5/SCK  (via drill 0.3)
  Top 0.254: v61.85,30.35 60.96,30.35 R12.1
  Bottom 0.254: U1.35 62.36,27.94 62.23,28.07 62.23,29.97 v61.85,30.35
PWDN  (via drill 0.3)
  Top 0.203: U$3.45 42.63,33.51 v42.86,33.27 42.86,33.08 43.31,32.64 43.69,32.64
  Top 0.254: R3.1 43.69,32.64
  Top 0.305: U6.3 v56.25,38.59
  Bottom 0.203: 42.99,33.15 v42.86,33.27
  Bottom 0.254: v56.25,38.59 51.67,38.59 46.23,33.15 42.99,33.15
PWDN1
  Top 0.406: J2.2 62.99,41.91 62.99,39.88 62.48,39.37 R27.1 R16.2
PWR_IN
  Top 0.61: U1.23 46.35,3.17 D1.-
RESET
  Top 0.406: 20.95,2.41 K1.P$2 | K1.P$2 22.48,2.92 24.38,1.02 31.5,1.02 U1.28 32.89,2.67 | D3.- 24,5.46 K1.P$2 | RST.- 20.57,2.03 K1.P$2
RX+  (via drill 0.3)
  Top 0.305: U4.6 23.5,15.37 21.08,17.78 13.84,17.78 13.72,17.91 v13.72,18.16 | J3.$3 13.07,22.87 v13.72,22.23
  Bottom 0.305: v13.72,22.23 v13.72,18.16
RX-
  Top 0.305: U4.8 26.04,16.38 23.37,19.05 13.46,19.05 12.7,19.81 12.69,19.81 J3.$6
RXIN
  Top 0.203: U$3.21 33.04,31.01 32.58,30.54 32.58,29.21 31.18,27.81 30.23,27.81 29.72,27.3 29.72,26.54 29.08,25.91 R23.1
  Top 0.305: U4.9 26.04,24.51 26.67,25.15 R23.1
RXIP
  Top 0.203: U$3.20 32.84,31.51 32,30.67 32,29.46 30.92,28.38 29.53,28.38 29.08,27.94 29.08,27.43 28.32,26.67 23.62,26.67 R22.2
  Top 0.305: U4.11 23.5,24.51 22.99,25.02 22.99,25.78 R22.2
SCK  (via drill 0.3)
  Top 0.203: U$3.42 41.65,32.01 43.81,29.84 v49.28,29.84
  Top 0.254: U2.6 55.4,30.38 v55.37,30.35
  Top 0.305: 57.15,23.5 54.61,26.04 54.61,29.59 v55.37,30.35
  Top 0.406: J1.5 56.26,13.97 57.15,14.86 57.15,23.5
  Bottom 0.203: v49.28,29.84 54.86,29.84 v55.37,30.35
SPD
  Top 0.254: U$3.31 37.59,28.2 37.72,28.07 40.13,28.07 40.77,27.43 42.1,27.43 R8.2 R9.1
SPDLED  (via drill 0.3)
  Top 0.203: U$3.4 38.59,36.47 36.96,38.1 36.96,41.15 36.7,41.4 36.7,42.04 v36.07,42.67
  Top 0.254: v19.56,40.01 SPDLED.-
  Bottom 0.203: 35.69,42.42 35.94,42.67 v36.07,42.67
  Bottom 0.254: v19.56,40.01 25.27,40.01 27.69,42.42 35.69,42.42
TCS  (via drill 0.3)
  Top 0.254: U2.11 v52.7,29.08
  Top 0.305: U2.1 56.04,27.08 56.01,27.05 v55.75,27.05
  Top 0.406: J1.2 50.67,17.14 53.59,17.14 54.48,18.03 v54.48,18.29
  Bottom 0.305: v52.7,29.08 54.74,27.05 | v55.75,27.05 54.74,27.05 | 54.74,27.05 54.61,26.92
  Bottom 0.406: v54.48,18.29 54.61,18.41 54.61,26.92
TFSS
  Top 0.254: U1.5 53.34,50.29 54.74,48.9 54.74,36.45 53.98,35.69 53.98,34.67 54.36,34.29 R13.1
TMISO
  Top 0.305: U2.2 57.12,27.75 58.04,27.75 58.42,27.37
  Top 0.406: J1.7 50.63,11.68 56.39,11.68 58.42,13.72 58.42,27.37
TX+  (via drill 0.3)
  Top 0.254: 17.14,13.72 17.4,13.46 17.4,13.75 U4.1
  Top 0.305: 10.51,24.89 J3.$1 13.57,24.91 v13.59,24.89 | v16.26,15.62 17.14,14.73 U4.1
  Bottom 0.305: v13.59,24.89 15.11,24.89 16.26,23.75 v16.26,15.62
TX-  (via drill 0.3)
  Top 0.305: U4.3 19.68,15.62 18.8,16.51 15.37,16.51 v14.86,17.02 | J3.$2 14.09,23.89 v14.86,23.11
  Bottom 0.305: v14.86,23.11 v14.86,17.02
TXON
  Top 0.203: U$3.18 32.95,32.51 31.56,31.11 31.56,29.78 30.67,28.89 26.35,28.89 24.77,30.48 22.1,30.48 21.34,29.72 21.34,27.3 R21.1
  Top 0.305: U4.14 19.68,25.65 R21.1
TXOP
  Top 0.203: U$3.17 32.56,33.01 31.05,31.5 31.05,29.97 30.61,29.53 26.73,29.53 25.15,31.11 16.51,31.11 14.99,29.59 14.99,26.99 R20.2
  Top 0.305: U4.16 17.14,23.5 15.88,24.77 R20.2
W!INT  (via drill 0.3)
  Top 0.203: U$3.40 41.38,31.01 44.2,28.19 v46.23,28.19
  Top 0.254: U6.5 55.9,39.89 55.5,39.5 55.5,36.07 v54.99,35.56
  Top 0.305: 55.24,35.81 v54.99,35.56
  Bottom 0.254: v54.99,35.56 52.32,35.56 46.23,29.46 v46.23,28.19
W!INT1
  Top 0.406: R25.2 61.28,41.59 60.33,42.55 59.05,42.55 58.17,43.43 J2.1
WCS  (via drill 0.3)
  Top 0.203: U$3.41 41.52,31.51 43.81,29.21 44.96,29.21 v45.09,29.08 | 52.32,36.32 v51.56,36.32
  Top 0.254: 52.32,36.32 52.96,36.96 52.96,39.24 52.9,39.31 | 52.9,39.31 52.32,39.88 51.57,39.88 U6.10 | U6.11 52.83,39.24 52.9,39.31
  Bottom 0.203: v51.56,36.32 51.44,36.2 51.44,35.69 45.09,29.34 v45.09,29.08
WMISO
  Top 0.203: U$3.44 41.92,33.01 43.81,31.11 48.01,31.11
  Top 0.254: U6.9 52.93,40.54 54.1,39.37 54.1,37.21 48.01,31.11
WRST  (via drill 0.3)
  Top 0.254: v28.83,9.27 28.83,6.22 28.07,5.46 D3.+ | U$3.46 41.76,34.01 v42.04,34.29 42.93,34.29 43.18,34.04 43.81,34.04 R2.1
  Bottom 0.254: v28.83,9.27 28.83,13.08 42.04,26.29 v42.04,34.29
WSS
  Top 0.61: U1.11 36.58,49.78 38.73,47.62 43.56,47.62 R15.1
X0
  Top 0.305: U$3.2 39.59,38.26 C3.2 R1.2 39.5,41.15 X1.2
X1
  Top 0.254: U$3.1 40.13,35.75 40.13,36.07 41.53,37.47 C2.2
  Top 0.305: C2.2 41.53,39.37 R1.1 41.02,40.39 42.55,41.91 42.55,42.42 X1.1
XTALVDD
  Top 0.254: C5.2 31.11,32.38 32.24,33.51 U$3.16
  Top 0.406: C5.2 30.35,31.62 29.84,31.11 29.84,30.8 C6.2

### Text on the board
tPlace: J2 | J1 | W!INT | PWDN | ICSP | J5 | J4
bPlace: Ethernet Shield | v1.2 2014/06/07 | www.elecrow.com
